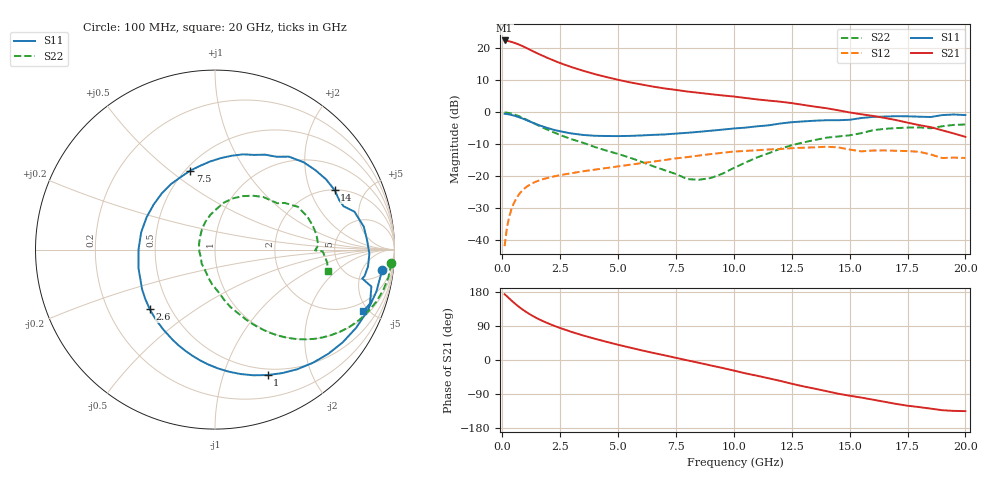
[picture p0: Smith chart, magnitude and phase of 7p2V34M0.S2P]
! Infineon Technologies  Discrete & RF Semiconductors
! bfp620
! VCE =  2.3 V,  IC =  4.0 mA
! Common Emitter S-Parameters:  Sep 2002
# GHz  S  MA  R  50
!  f  S11  S21  S12  S22
! GHz  MAG  ANG  MAG  ANG  MAG  ANG  MAG  ANG
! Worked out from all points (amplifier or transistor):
!   59 points, 100 MHz to 20 GHz, reference 50 ohm
!   highest |S21| = 22.3 dB at 100 MHz (marker M1)
!   |S21| within 3 dB of that: start of sweep to 1.226 GHz
!   unconditionally stable (mu >= 1): 5.008 GHz to 11.94 GHz; 14.55 GHz to 15.44 GHz; 17.3 GHz to end of sweep
!   at 1 GHz: K = 0.28, MSG = 21.9 dB, |S12| = -23.6 dB
!   at 5.5 GHz: K = 1.04, MAG = 11.7 dB, |S12| = -16.5 dB
!   at 20 GHz: K = 1.31, MAG = 0.0 dB, |S12| = -14.3 dB
!   S11 on the Smith chart (normalised r, x): 100 MHz: 7, -13; 1 GHz: 0.43, -1.42; 2.6 GHz: 0.38, -0.34; 7.5 GHz: 0.53, +0.59; 14 GHz: 2.02, +3.00; 20 GHz: 1.35, -4.65
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0.1  0.9378 -7.1  13.05 173.6  0.0081 72.1  0.9852 -4.5
0.3  0.9159 -21.8  12.65 162.4  0.0234 76.1  0.9645 -13.5
0.5  0.8795 -35.9  12.05 151.4  0.038 69.6  0.9216 -21.9
0.6  0.8576 -42.6  11.71 146.2  0.0446 66.3  0.895 -25.9
0.8  0.8092 -55.4  10.95 136.6  0.0564 59.9  0.8362 -33.0
1  0.758 -67.2  10.13 128.0  0.0661 54.2  0.7741 -39.2
1.4  0.6625 -88.5  8.603 113.4  0.0806 45.2  0.6567 -49.0
1.7  0.6035 -102.3  7.657 104.2  0.0884 40.2  0.5828 -54.5
2.2  0.5308 -122.8  6.401 91.2  0.0984 34.1  0.4858 -61.6
2.6  0.4922 -137.7  5.619 82.2  0.1053 30.5  0.4245 -66.2
3  0.4629 -151.3  4.997 73.9  0.1114 27.3  0.376 -70.2
3.5  0.4386 -166.4  4.39 64.6  0.1193 24.1  0.3305 -75.0
5  0.4214 154.7  3.179 40.2  0.1421 15.6  0.2221 -88.1
7  0.4469 115.2  2.334 12.5  0.1781 3.9  0.1243 -117.5
7.5  0.4611 107.5  2.21 5.7  0.1894 0.2  0.108 -133.4
9  0.5107 86.4  1.898 -14.3  0.2205 -11.6  0.0936 161.9
10.5  0.571 67.5  1.656 -35.2  0.2476 -26.6  0.1628 109.5
12  0.6617 51.5  1.449 -55.1  0.2645 -40.1  0.2671 79.1
13.5  0.7323 32.3  1.213 -75.7  0.2816 -55.7  0.3662 55.1
14  0.7445 26.4  1.146 -82.2  0.2875 -61.8  0.3978 47.5
17  0.8604 -1.5  0.75 -115.8  0.2487 -86.6  0.561 13.6
20  0.8954 -22.5  0.41 -134.9  0.1921 -102.0  0.6382 -10.7
